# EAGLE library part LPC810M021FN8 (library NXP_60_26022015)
32-bit ARM Cortex-M0+ microcontroller The LPC81xM are an ARM Cortex-M0+ based, low-cost 32-bit MCU family operating at CPU frequencies of up to 30 MHz. The LPC81xM support up to 16 kB of flash memory and 4 kB of SRAM. The peripheral complement of the LPC81xM includes a CRC engine, one I 2 C-bus interface, up to three USARTs, up to two SPI interfaces, one multi-rate timer, self wake-up timer, and state-configurable timer, one comparator, function-configurable I/O ports through a switch matrix, an input pattern match engine, and up to 18 general-purpose I/O pins. AAL Eindhoven MK
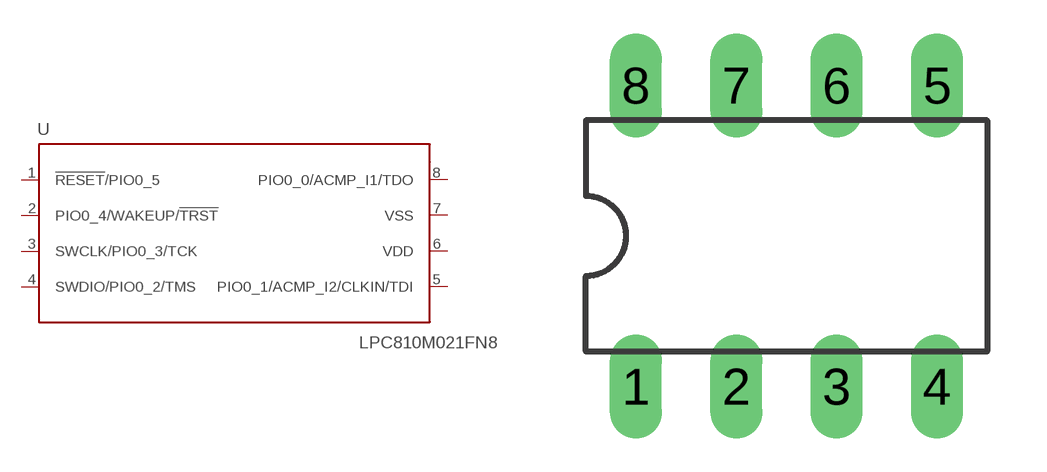
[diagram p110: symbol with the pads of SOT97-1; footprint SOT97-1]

Designator prefix U

## LPC810M021FN8 (COMP: 1; FLASH: 4k; GPIO: 6; I2C: 1; SPI: 1; SRAM: 1k; USART: 2)  [SOT97-1]
1  !RESET!/PIO0_5
2  PIO0_4/WAKEUP/!TRST!
3  SWCLK/PIO0_3/TCK
4  SWDIO/PIO0_2/TMS
5  PIO0_1/ACMP_I2/CLKIN/TDI
6  VDD  pwr
7  VSS  pwr
8  PIO0_0/ACMP_I1/TDO

## Footprint SOT97-1 (pad centres in mm)
Dual In Line Package
drill 0.813 long: 1 -3.81,-3.81; 2 -1.27,-3.81; 3 1.27,-3.81; 4 3.81,-3.81; 5 3.81,3.81; 6 1.27,3.81; 7 -1.27,3.81; 8 -3.81,3.81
